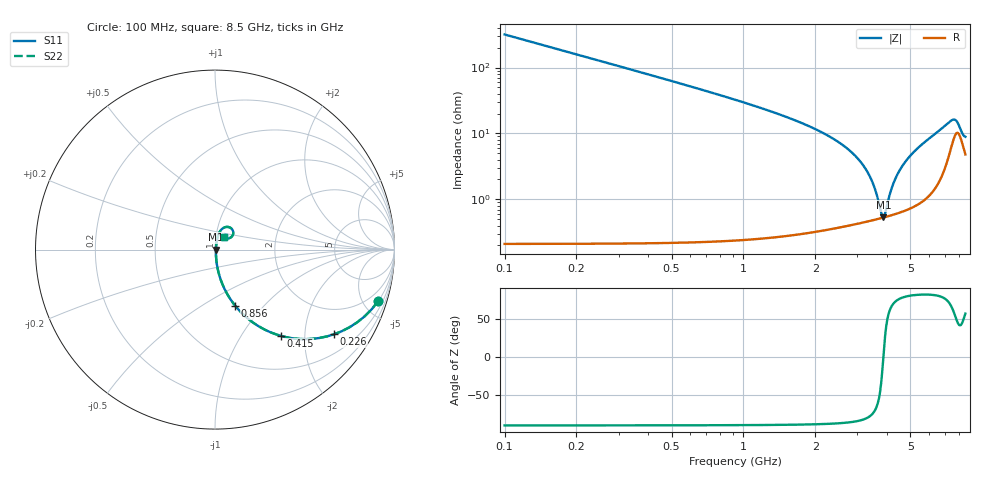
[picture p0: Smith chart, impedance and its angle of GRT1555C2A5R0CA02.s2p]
!Murata Part Number: GRT1555C2A5R0CA02
!These Parameters are Measured in Series Mode Connection
!Data Generated on Jun 19, 2026
!  o--ll--o
!Port1  Port2
!  o------o
!Operation Temp=25[degC], DC Bias Voltage=0[V]
!Freq. Start=100[MHz] Stop=9[GHz] 401[Steps]
# Hz S RI R 50
!Freq.(Hz) S11(Real) S11(Imag) S21(Real) S21(Imag) S12(Real) S12(Imag) S22(Real) S22(Imag)
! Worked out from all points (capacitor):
!   401 points, 100 MHz to 8.5 GHz, reference 50 ohm
!   read as one part in series: C = 5 pF near 142 MHz
!   lowest |Z| = 530 mohm at 3.859 GHz (marker M1)
!   series resonance near 3.854 GHz, so ESL is about 340 pH
!   S11 on the Smith chart (normalised r, x): 100 MHz: 1.00, -6.36; 226 MHz: 1.00, -2.81; 415 MHz: 1.00, -1.52; 856 MHz: 1.00, -0.71; 8.5 GHz: 1.10, +0.15
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1e8  0.9099 -0.286  0.0901 0.286  0.0901 0.286  0.9099 -0.286
2.26e8  0.6631 -0.4719  0.3369 0.4719  0.3369 0.4719  0.6631 -0.4719
4.15e8  0.3653 -0.4801  0.6347 0.4801  0.6347 0.4801  0.3653 -0.4801
6.04e8  0.21 -0.4052  0.79 0.4052  0.79 0.4052  0.21 -0.4052
8.56e8  0.1127 -0.3129  0.8873 0.3129  0.8873 0.3129  0.1127 -0.3129
1.507e9  0.0335 -0.1725  0.9665 0.1725  0.9665 0.1725  0.0335 -0.1725
2.914e9  0.00631 -0.0465  0.9937 0.0465  0.9937 0.0465  0.00631 -0.0465
3.187e9  0.00544 -0.0315  0.9946 0.0315  0.9946 0.0315  0.00544 -0.0315
3.418e9  0.00511 -0.0199  0.9949 0.0199  0.9949 0.0199  0.00511 -0.0199
3.586e9  0.00506 -0.0119  0.9949 0.0119  0.9949 0.0119  0.00506 -0.0119
3.796e9  0.00519 -0.0025  0.9948 0.0025  0.9948 0.0025  0.00519 -0.0025
3.859e9  0.00527 0.000229  0.9947 -0.000229  0.9947 -0.000229  0.00527 0.000229
3.922e9  0.00536 0.00292  0.9946 -0.00292  0.9946 -0.00292  0.00536 0.00292
4.132e9  0.00578 0.0116  0.9942 -0.0116  0.9942 -0.0116  0.00578 0.0116
4.3e9  0.00623 0.0184  0.9938 -0.0184  0.9938 -0.0184  0.00623 0.0184
4.531e9  0.00702 0.0273  0.993 -0.0273  0.993 -0.0273  0.00702 0.0273
4.846e9  0.00841 0.0391  0.9916 -0.0391  0.9916 -0.0391  0.00841 0.0391
5.707e9  0.0146 0.0702  0.9854 -0.0702  0.9854 -0.0702  0.0146 0.0702
7.114e9  0.0511 0.1229  0.9489 -0.1229  0.9489 -0.1229  0.0511 0.1229
7.702e9  0.0988 0.1075  0.9012 -0.1075  0.9012 -0.1075  0.0988 0.1075
8.269e9  0.0682 0.0622  0.9318 -0.0622  0.9318 -0.0622  0.0682 0.0622
8.5e9  0.0507 0.0679  0.9493 -0.0679  0.9493 -0.0679  0.0507 0.0679
